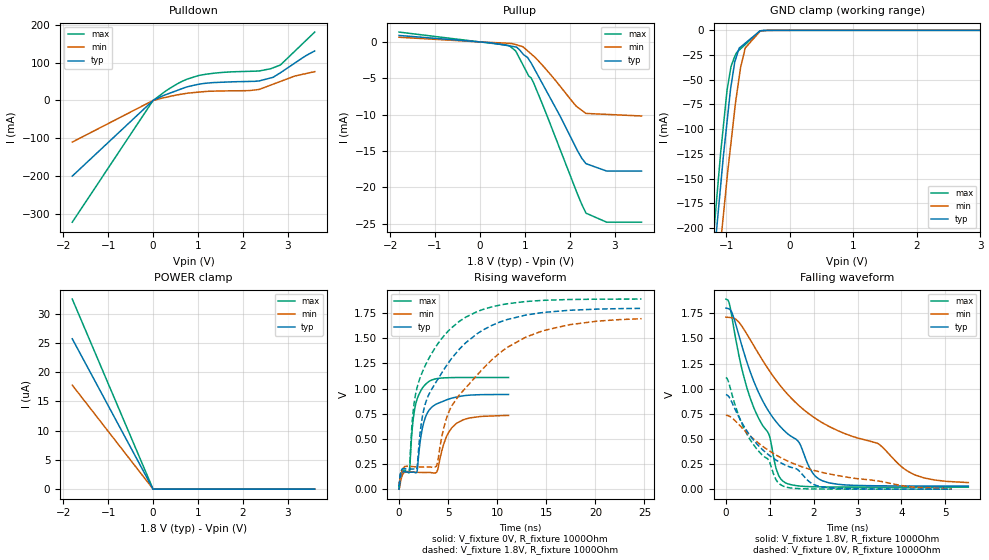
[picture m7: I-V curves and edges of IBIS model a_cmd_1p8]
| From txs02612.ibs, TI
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|   a_cmd_1p8 Model
[Model]   a_cmd_1p8
Model_type   I/O
Polarity   Non-Inverting
Enable   Active-High
Vinl = 0.15
Vinh = 1.6
Vmeas = 0.9
Vref = 0.9
Cref = 2pF
Rref = 1000
|   typ   min   max
|   (nom PVT)   (fast PVT)   (slow PVT)
|C_comp from frequency sweep method (F=30MHz)
C_comp   6.024e-12   5.939e-12   6.112e-12
|ON state : BUFFER OUTPUT TURNED HIGH
|C_comp   5.776e-12   5.357e-12   6.444e-12
|OFF state: BUFFER IN HIGH IMPEDANCE
|C_comp   6.024e-12   5.939e-12   6.112e-12
|C_comp from LC tank measurement(L=1nH)
|Average
|Resonant Frequency(Hz)   2.285e+09   2.325e+09   2.270e+09
|C_comp   4.857e-12   4.690e-12   4.921e-12
|ON state : BUFFER OUTPUT TURNED HIGH
|Resonant Frequency(Hz)   2.280e+09   2.320e+09   2.270e+09
|C_comp   4.878e-12   4.711e-12   4.921e-12
|OFF state: BUFFER IN HIGH IMPEDANCE
|Resonant Frequency(Hz)   2.290e+09   2.330e+09   2.270e+09
|C_comp   4.835e-12   4.670e-12   4.921e-12
[Model spec]
|subparameter
Vinl   0.15   0.15   0.15
Vinh   1.6   1.51   1.69
| Where nom  PVT is Nominal Process, 1.8V, 27C
|   Fast PVT is Strong Process,  1.89V, -40C
|   Slow PVT is Weak Process,   1.71V, 125C
[Voltage Range]   1.8   1.71   1.89
|Ambient Temperature   25   85   -40
|Junction Temperature
[Temperature Range]   27   125   -40
[Pullup Reference]   1.8   1.71   1.89
[Pulldown Reference]   0   0   0
[Power Clamp Reference]   1.8   1.71   1.89
[GND Clamp Reference]   0   0   0
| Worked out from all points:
|   slope of the pulldown table from 0 to 0.27 V, typ, clamps not added: 18.4 ohm
|   slope of the pullup table from 0 to 0.27 V, typ, clamps not added: 1.95 kohm
|   GND clamp passes 1 mA (typ) near -0.48 V on its own axis
|   falling waveform, V_fixture 1.8V, R_fixture 1000Ohm: 20-80 % time 1.4ns typ, 2.92ns min, 842ps max; typ from 1.8 V to 0.032 V
|   rising waveform, V_fixture 0V, R_fixture 1000Ohm: 20-80 % time 1.01ns typ, 4.84ns min, 707ps max; typ from 0.002 V to 0.942 V
|   rising waveform, V_fixture 1.8V, R_fixture 1000Ohm: 20-80 % time 4.7ns typ, 6.31ns min, 3.33ns max; typ from 0.032 V to 1.8 V
|   falling waveform, V_fixture 0V, R_fixture 1000Ohm: 20-80 % time 1.4ns typ, 1.95ns min, 859ps max; typ from 0.942 V to 0.002 V
[Pulldown]
|   Voltage   I(typ)   I(min)   I(max)
-1.8V     -199.5mA   -109.8mA   -321mA
0V        0A         0A         0A
525.4mV   25.9mA     14.28mA    42.84mA
754.1mV   35.71mA    18.9mA     56.06mA
1.011V    42.5mA     21.91mA    65.62mA
1.542V    48.08mA    25.01mA    73.87mA
2.146V    50.16mA    26.02mA    76.8mA
2.362V    51.49mA    29.01mA    77.69mA
2.673V    60.98mA    42.83mA    86.08mA
2.835V    72.9mA     50.04mA    93.35mA
3.158V    98.68mA    64.44mA    130.1mA
3.6V      130.5mA    75.95mA    180.2mA
[GND Clamp]
|   Voltage   I(typ)   I(min)   I(max)
-1.8V     -683.8mA   -700.8mA   -693mA
-1.213V   -241.9mA   -295.6mA   -215mA
-1.153V   -199.6mA   -253.7mA   -169.5mA
-1.092V   -157.7mA   -215.1mA   -124.5mA
-1.049V   -127.7mA   -187.5mA   -97.39mA
-988.5mV  -91.09mA   -148.3mA   -59.51mA
-928mV    -56.21mA   -113.2mA   -36.54mA
-869.4mV  -32mA      -79.73mA   -26.26mA
-778.1mV  -16.89mA   -37.86mA   -18.74mA
-704.5mV  -12.98mA   -17.87mA   -14.38mA
-470.6mV  -590.8uA   -935.7uA   -502.6uA
3.6V      0A         0A         0A
[Pullup]
|   Voltage   I(typ)   I(min)   I(max)
-1.8V     890.7uA    643.4uA    1.354mA
252mV     -119.8uA   -71.93uA   -184.4uA
655.8mV   -541uA     -202.3uA   -524.1uA
817.2mV   -709.3uA   -394.2uA   -1.473mA
957.6mV   -1.645mA   -667.9uA   -3.144mA
1.085V    -2.361mA   -1.346mA   -4.665mA
1.139V    -2.872mA   -1.639mA   -4.954mA
1.461V    -6.515mA   -3.687mA   -9.627mA
2.153V    -14.72mA   -8.883mA   -20.62mA
2.364V    -16.76mA   -9.846mA   -23.58mA
2.824V    -17.78mA   -9.976mA   -24.82mA
3.6V      -17.78mA   -10.2mA    -24.82mA
[POWER Clamp]
|   Voltage   I(typ)   I(min)   I(max)
-1.8V     25.72uA    17.79uA    32.51uA
-68.4mV   978.3nA    697.9nA    1.238uA
-37.97fV  0A         0A         0A
3.6V      0A         0A         0A
[Ramp]
R_load = 1000
|   typ   min   max
dV/dt_r   0.564173/1.00695e-09  0.441121/4.84032e-09   0.665318/7.07204e-10
dV/dt_f   1.06074/1.39798e-09   0.992686/2.94209e-09   1.12116/8.42406e-10
[Falling Waveform]
V_fixture = 1.8V
V_fixture_min = 1.71V
V_fixture_max = 1.89V
R_fixture = 1000Ohm
|   Time   V(typ)   V(min)   V(max)
0s        1.8V       1.71V      1.89V
150ps     1.741V     1.703V     1.68V
500ps     1.236V     1.526V     978.5mV
975ps     775.3mV    1.188V     551.6mV
1.15ns    668.5mV    1.08V      198.5mV
1.3ns     595.4mV    997.7mV    81.55mV
2.35ns    64.4mV     624.9mV    23.52mV
3.45ns    35.22mV    458.9mV    21.79mV
4.325ns   33.26mV    140.6mV    21.52mV
5.525ns   32.49mV    67.71mV    21.42mV
[Rising Waveform]
V_fixture = 0V
V_fixture_min = 0V
V_fixture_max = 0V
R_fixture = 1000Ohm
|   Time   V(typ)   V(min)   V(max)
0s        1.904mV    2.084mV    1.826mV
225ps     154.7mV    107.4mV    165mV
1.05ns    170.7mV    175.4mV    168mV
1.4ns     171.1mV    171.8mV    662.3mV
1.8ns     169.6mV    169.2mV    885.5mV
2.675ns   713.4mV    167.2mV    1.041V
3.825ns   848mV      171.1mV    1.099V
4.8ns     887.2mV    516.6mV    1.108V
5.9ns     918.1mV    658.8mV    1.11V
11.15ns   942.1mV    734mV      1.111V
[Rising Waveform]
V_fixture = 1.8V
V_fixture_min = 1.71V
V_fixture_max = 1.89V
R_fixture = 1000Ohm
|   Time   V(typ)   V(min)   V(max)
0s        32.11mV    55.52mV    21.4mV
1.05ns    201.5mV    229.4mV    190.6mV
1.475ns   202.5mV    225.3mV    813.3mV
1.825ns   215.1mV    223.3mV    1.007V
2.125ns   544.5mV    222.3mV    1.104V
3.8ns     1.071V     229.7mV    1.425V
4.8ns     1.224V     697.6mV    1.55V
6.1ns     1.388V     934mV      1.666V
13.03ns   1.733V     1.516V     1.866V
24.7ns    1.797V     1.695V     1.89V
[Falling Waveform]
V_fixture = 0V
V_fixture_min = 0V
V_fixture_max = 0V
R_fixture = 1000Ohm
|   Time   V(typ)   V(min)   V(max)
0s        942.2mV    737.3mV    1.111V
450ps     599.3mV    573.6mV    572.8mV
700ps     454mV      474.6mV    403.4mV
975ps     342.4mV    386.3mV    289.3mV
1.125ns   296.2mV    345.6mV    110.9mV
1.275ns   258.4mV    309.7mV    38.89mV
1.625ns   199.4mV    241.2mV    8.276mV
2ns       48.87mV    188.6mV    4.102mV
2.275ns   18.44mV    160.3mV    3.179mV
5.15ns    2.183mV    6.656mV    1.847mV
